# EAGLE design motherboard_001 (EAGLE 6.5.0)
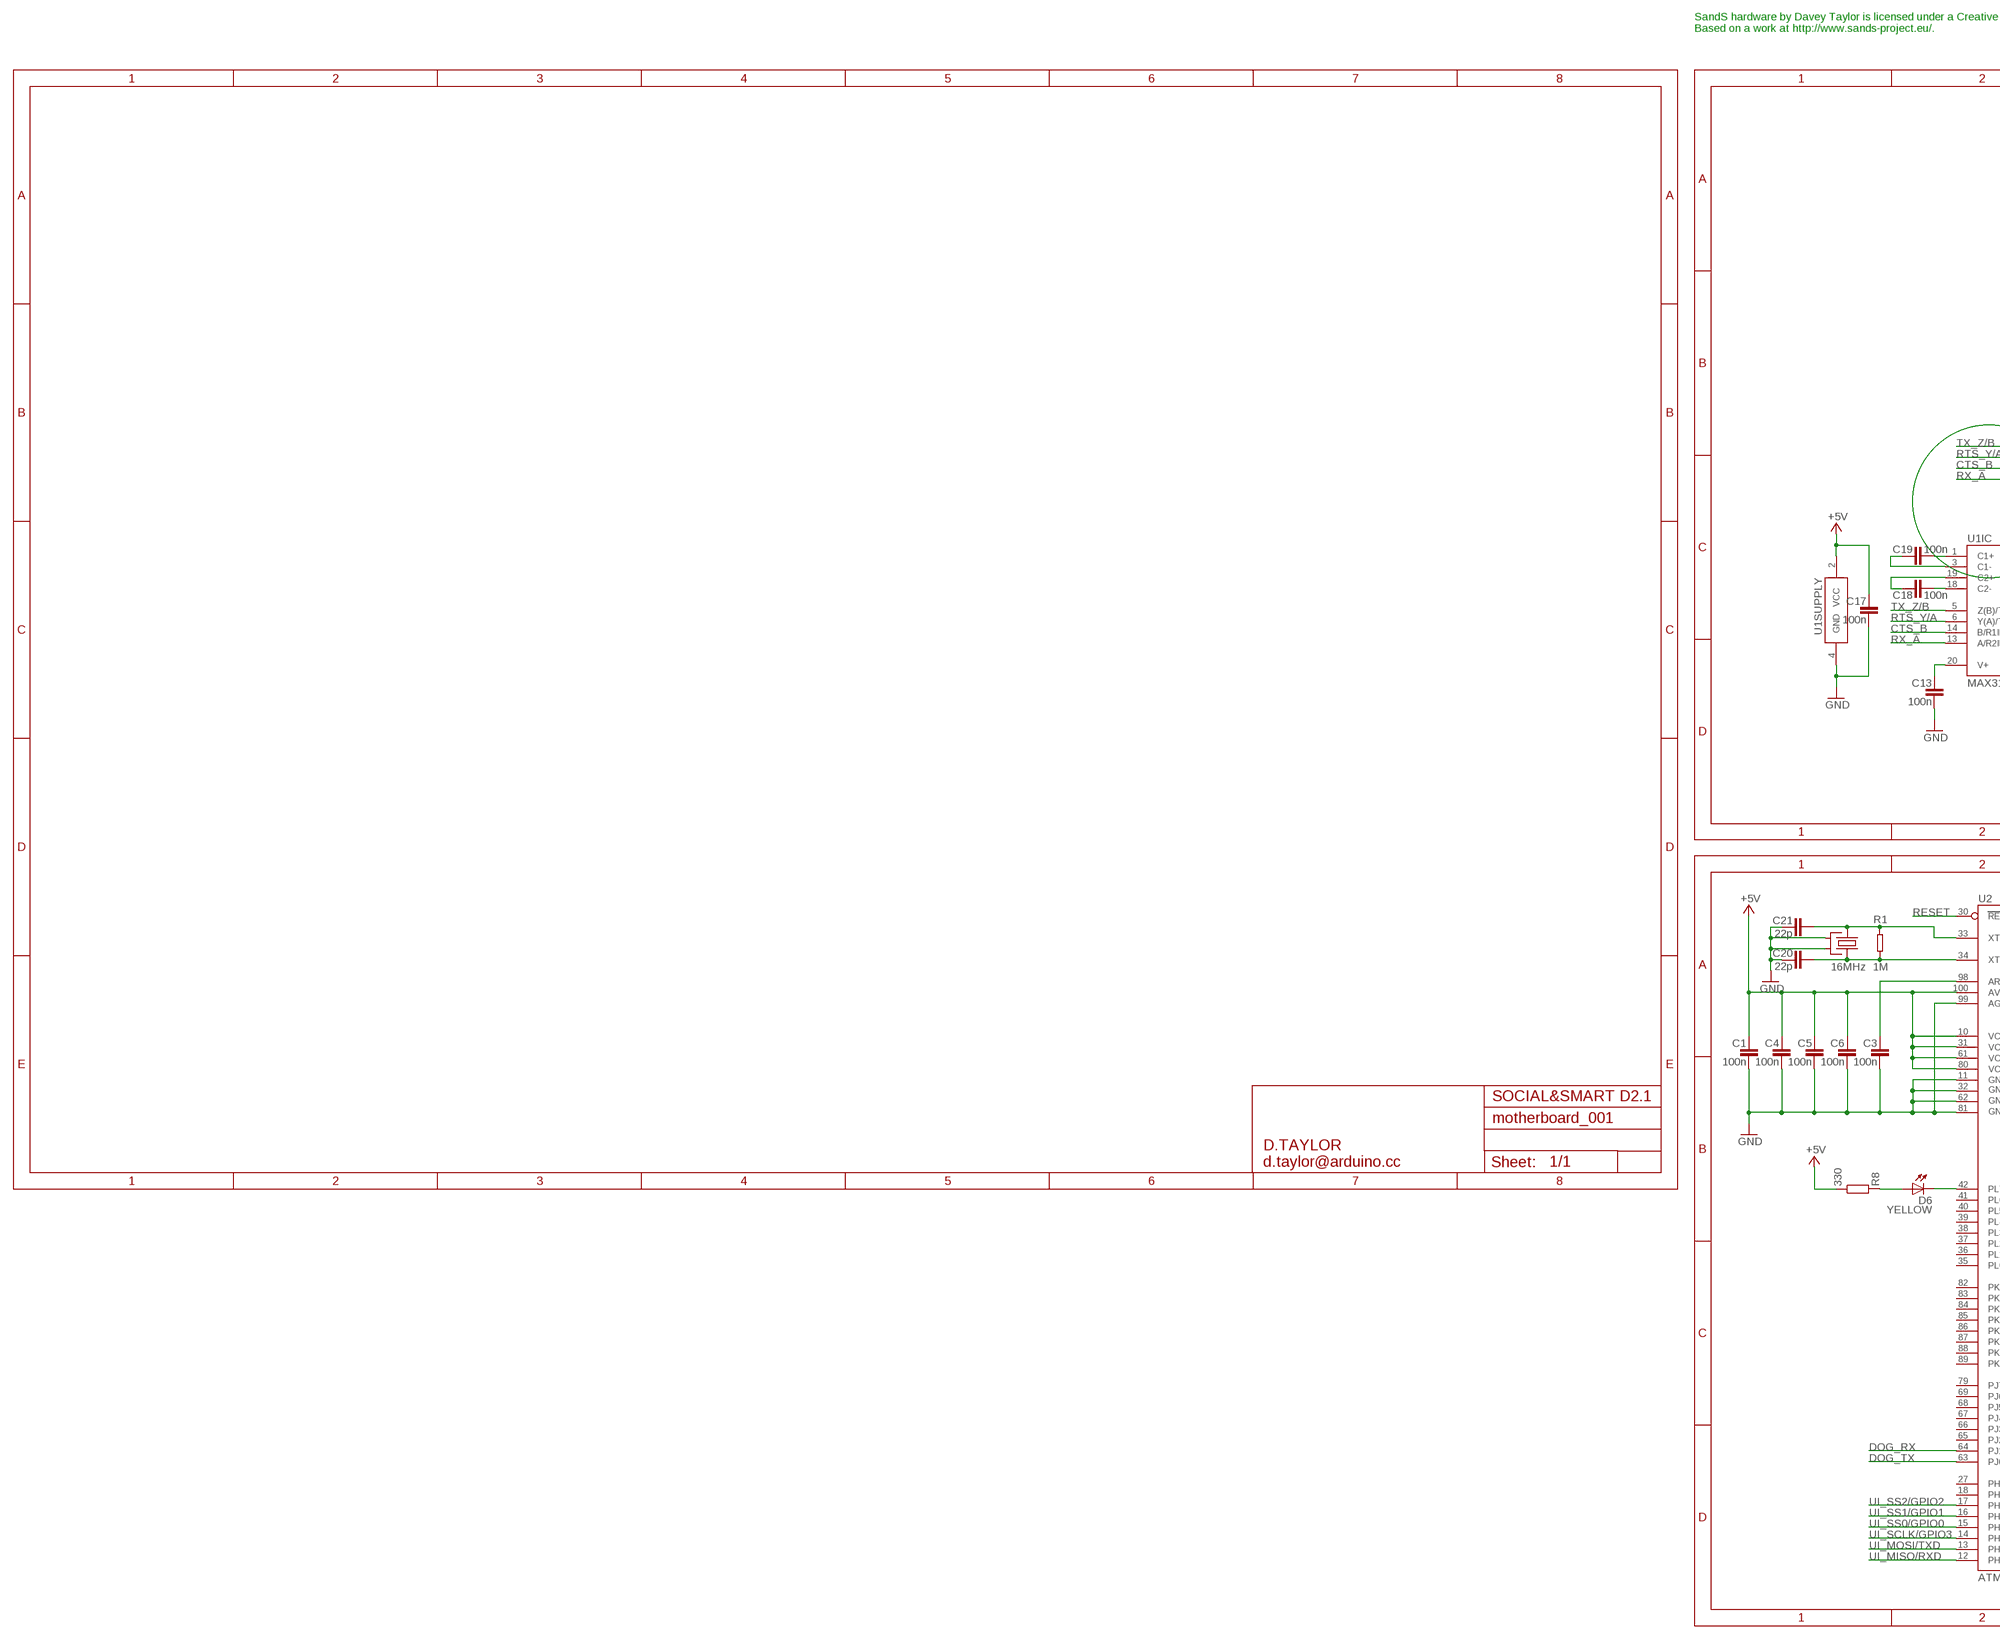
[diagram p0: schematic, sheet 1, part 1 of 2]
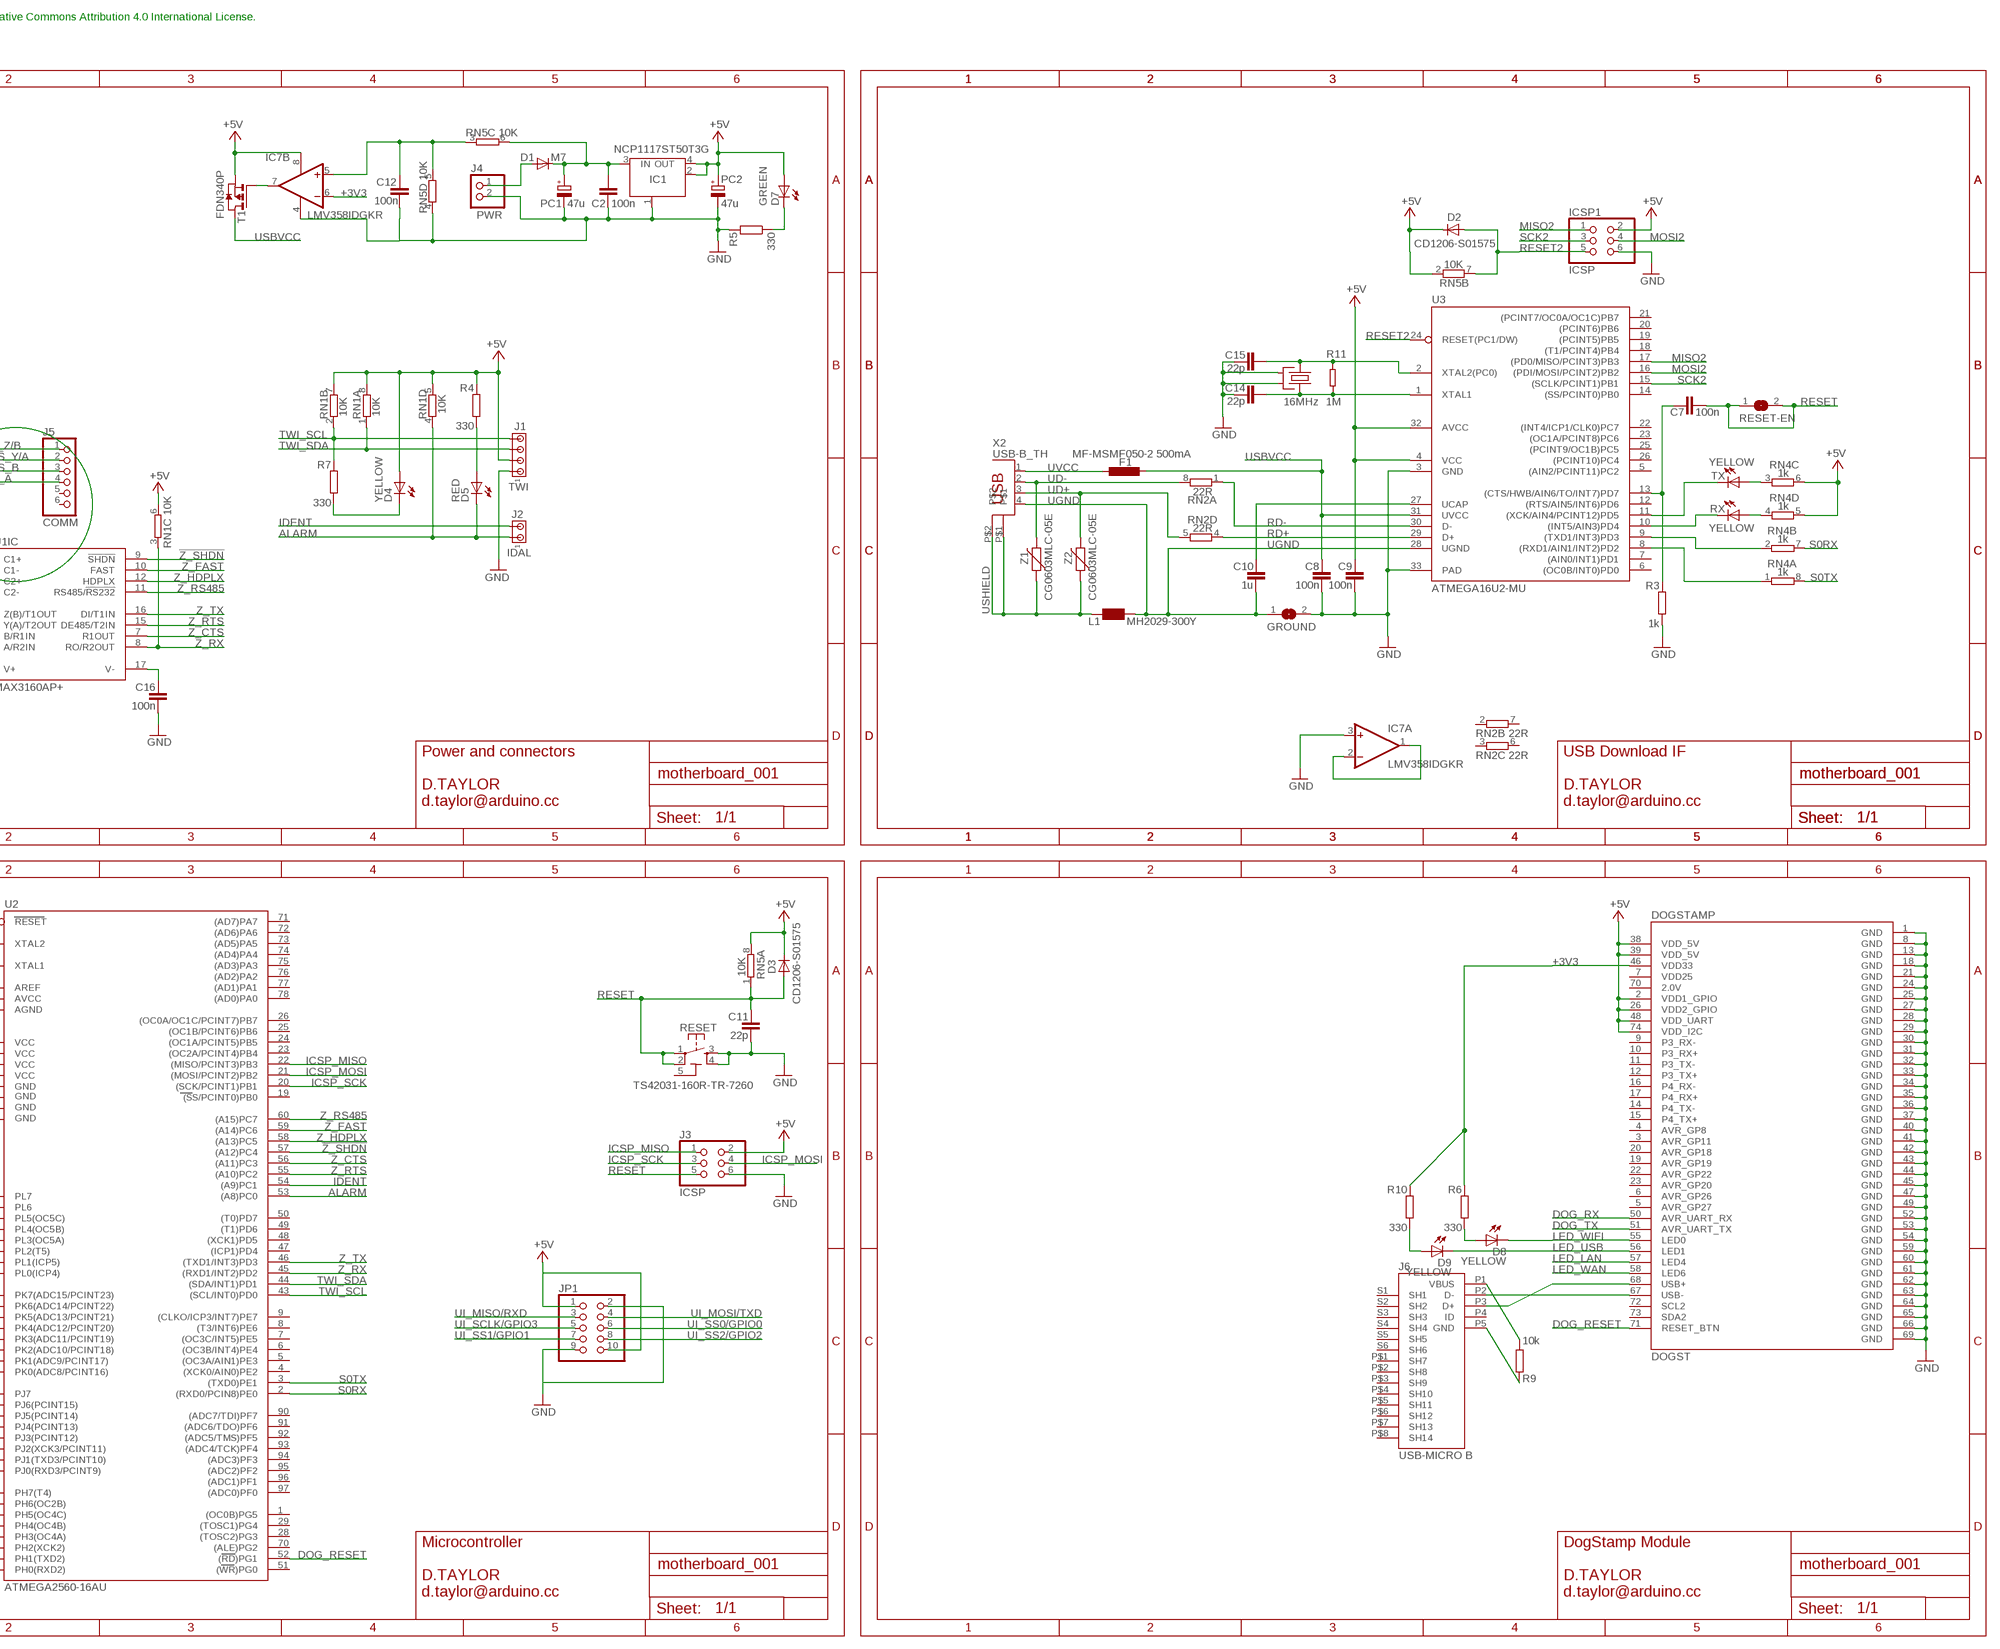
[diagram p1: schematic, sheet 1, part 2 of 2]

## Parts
C1  100n  C-EU0603-RND  [C0603-ROUND]
C2  100n  C-EU0603-RND  [C0603-ROUND]
C3  100n  C-EU0603-RND  [C0603-ROUND]
C4  100n  C-EU0603-RND  [C0603-ROUND]
C5  100n  C-EU0603-RND  [C0603-ROUND]
C6  100n  C-EU0603-RND  [C0603-ROUND]
C7  100n  C-EU0603-RND  [C0603-ROUND]
C8  100n  C-EU0603-RND  [C0603-ROUND]
C9  100n  C-EU0603-RND  [C0603-ROUND]
C10  1u  C-EU0603-RND  [C0603-ROUND]
C11  22p  C-EU0603-RND  [C0603-ROUND]
C12  100n  C-EU0603-RND  [C0603-ROUND]
C13  100n  C-EU0603-RND  [C0603-ROUND]
C14  22p  C-EU0603-RND  [C0603-ROUND]
C15  22p  C-EU0603-RND  [C0603-ROUND]
C16  100n  C-EU0603-RND  [C0603-ROUND]
C17  100n  C-EU0603-RND  [C0603-ROUND]
C18  100n  C-EU0603-RND  [C0603-ROUND]
C19  100n  C-EU0603-RND  [C0603-ROUND]
C20  22p  C-EU0603-RND  [C0603-ROUND]
C21  22p  C-EU0603-RND  [C0603-ROUND]
D1  M7  DIODE-SMB  [SMB]
D2  CD1206-S01575  DIODE-MINIMELF  [MINIMELF]
D3  CD1206-S01575  DIODE-MINIMELF  [MINIMELF]
D4  YELLOW  LEDCHIP-LED0805  [CHIP-LED0805]
D5  RED  LEDCHIP-LED0805  [CHIP-LED0805]
D6  YELLOW  LEDCHIP-LED0805  [CHIP-LED0805]
D7  GREEN  LEDCHIP-LED0805  [CHIP-LED0805]
D8  YELLOW  LEDCHIP-LED0805  [CHIP-LED0805]
D9  YELLOW  LEDCHIP-LED0805  [CHIP-LED0805]
DOGSTAMP  DOGST  [DOGST]
F1  MF-MSMF050-2 500mA  L-EUL1812  [L1812]
GROUND  SJ  [SJ]
IC1  NCP1117ST50T3G  MC33269ST-3.3T3  [SOT223]
IC7  LMV358IDGKR  LMV358MMX  [MSOP08]
ICSP1  ICSP  PINHD-2X3  [2X03]
J1  TWI  MTA04-100  [10X04MTA]
J2  IDAL  MTA02-100  [10X02MTA]
J3  ICSP  PINHD-2X3  [2X03]
J4  PWR  MKDS_1,5/2-5,08  [MKDS1,5/2-5,08]
J5  COMM  PINHD-1X6  [1X06]
J6  USB-MICRO B  MYCON2_USB-MINI-B  [CON2_USB_MICRO_B_AT]
JP1  PINHD-2X5  [2X05]
L1  MH2029-300Y  WE-CBF_0805  [0805]
PC1  47u  CPOL-EUD  [PANASONIC_D]
PC2  47u  CPOL-EUD  [PANASONIC_D]
R1  1M  R-EU_0603-RND  [R0603-ROUND]
R3  1k  R-EU_R0603  [R0603-ROUND]
R4  330  R-EU_R0603  [R0603-ROUND]
R5  330  R-EU_R0603  [R0603-ROUND]
R6  330  R-EU_R0603  [R0603-ROUND]
R7  330  R-EU_R0603  [R0603-ROUND]
R8  330  R-EU_R0603  [R0603-ROUND]
R9  10k  R-EU_R0603  [R0603-ROUND]
R10  330  R-EU_R0603  [R0603-ROUND]
R11  1M  R-EU_0603-RND  [R0603-ROUND]
RESET  TS42031-160R-TR-7260  TS42  [TS42]
RESET-EN  SJ  [SJ]
RN1  10K  4R-NCAT16  [CAT16]
RN2  22R  4R-NCAY16  [CAY16]
RN4  1k  4R-NCAY16  [CAY16]
RN5  10K  4R-NCAT16  [CAT16]
RX  YELLOW  LEDCHIP-LED0805  [CHIP-LED0805]
T1  FDN340P  PMOSSOT23  [SOT-23]
TX  YELLOW  LEDCHIP-LED0805  [CHIP-LED0805]
U1  MAX3160AP+  [SSOP20(G)]
U2  ATMEGA2560-16AU  ATMEGA25602560-16AU  [TQFP100]
U3  ATMEGA16U2-MU  [MLF32]
X1  16MHz  CRYSTAL2-KX7  [XTAL-3.2-2.5]
X2  USB-B_TH  PN61729  [PN61729]
X3  16MHz  CRYSTAL2-KX7  [XTAL-3.2-2.5]
Z1  CG0603MLC-05E  VARISTORCN0603  [CT/CN0603]
Z2  CG0603MLC-05E  VARISTORCN0603  [CT/CN0603]

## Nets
!Z_SHDN!: U1.9(IC:!SHDN!) U2.57((A12)PC4)
+3V3 [power]: DOGSTAMP.46(VDD33) IC7.6(B:-IN) R6.2 R10.2
+5V: C1.1 C4.1 C5.1 C6.1 C9.1 C17.1 D2.C D3.C D4.A D7.A DOGSTAMP.2(VDD1_GPIO) DOGSTAMP.26(VDD2_GPIO) DOGSTAMP.38(VDD_5V) DOGSTAMP.39(VDD_5V) DOGSTAMP.48(VDD_UART) DOGSTAMP.74(VDD_I2C) IC1.2(OUT) IC1.4(OUT) IC7.8(P:V+) ICSP1.2 J1.2 J3.2 JP1.1 JP1.10 PC2.+ R4.2 R8.1 RN1.5 RN1.6 RN1.7 RN1.8 RN4.5 RN4.6 RN5.2 RN5.8 T1.2(S) U1.2(SUPPLY:VCC) U2.10(VCC) U2.31(VCC1) U2.61(VCC2) U2.80(VCC3) U2.100(AVCC) U3.4(VCC) U3.32(AVCC)
ALARM: D5.C J2.1 RN1.4 U2.53((A8)PC0)
CMP: C12.2 IC7.5(B:+IN) RN5.3 RN5.5
CTS_B: J5.3 U1.14(IC:B/R1IN)
DOG_RESET: DOGSTAMP.71(RESET_BTN) U2.52((RD)PG1)
DOG_RX: DOGSTAMP.50(AVR_UART_RX) U2.64(PJ1(TXD3/PCINT10))
DOG_TX: DOGSTAMP.51(AVR_UART_TX) U2.63(PJ0(RXD3/PCINT9))
DTR: C7.1 R3.2 U3.13((CTS/HWB/AIN6/TO/INT7)PD7)
GATE_CMD: IC7.7(B:OUT) T1.3(G)
GND: C1.2 C2.2 C3.2 C4.2 C5.2 C6.2 C8.2 C9.2 C11.2 C12.1 C13.2 C14.2 C15.2 C16.2 C17.2 C20.2 C21.2 DOGSTAMP.1(GND) DOGSTAMP.8(GND) DOGSTAMP.13(GND) DOGSTAMP.18(GND) DOGSTAMP.21(GND) DOGSTAMP.24(GND) DOGSTAMP.25(GND) DOGSTAMP.27(GND) DOGSTAMP.28(GND) DOGSTAMP.29(GND) DOGSTAMP.30(GND) DOGSTAMP.31(GND) DOGSTAMP.32(GND) DOGSTAMP.33(GND) DOGSTAMP.34(GND) DOGSTAMP.35(GND) DOGSTAMP.36(GND) DOGSTAMP.37(GND) DOGSTAMP.40(GND) DOGSTAMP.41(GND) DOGSTAMP.42(GND) DOGSTAMP.43(GND) DOGSTAMP.44(GND) DOGSTAMP.45(GND) DOGSTAMP.47(GND) DOGSTAMP.49(GND) DOGSTAMP.52(GND) DOGSTAMP.53(GND) DOGSTAMP.54(GND) DOGSTAMP.59(GND) DOGSTAMP.60(GND) DOGSTAMP.61(GND) DOGSTAMP.62(GND) DOGSTAMP.63(GND) DOGSTAMP.64(GND) DOGSTAMP.65(GND) DOGSTAMP.66(GND) DOGSTAMP.69(GND) GROUND.2 IC1.1(GND/ADJ) IC7.3(A:+IN) IC7.4(P:V-) ICSP1.6 J1.1 J3.6 J4.2 JP1.2 JP1.9 PC1.- PC2.- R3.1 R5.2 RESET.3 RESET.4 RN5.4 U1.4(SUPPLY:GND) U2.11(GND) U2.32(GND1) U2.62(GND2) U2.81(GND3) U2.99(AGND) U3.3(GND) U3.33(PAD) X1.2(SH1) X1.4(SH2) X3.2(SH1) X3.4(SH2)
ICSP_MISO: J3.1 U2.22((MISO/PCINT3)PB3)
ICSP_MOSI: J3.4 U2.21((MOSI/PCINT2)PB2)
ICSP_SCK: J3.3 U2.20((SCK/PCINT1)PB1)
IDENT: J2.2 U2.54((A9)PC1)
LED_LAN: DOGSTAMP.57(LED4)
LED_USB: D9.C DOGSTAMP.56(LED1)
LED_WAN: DOGSTAMP.58(LED6)
LED_WIFI: D8.C DOGSTAMP.55(LED0)
M8RXD: RN4.2 U3.9((TXD1/INT3)PD3)
M8TXD: RN4.1 U3.8((RXD1/AIN1/INT2)PD2)
MISO2: ICSP1.1 U3.17((PD0/MISO/PCINT3)PB3)
MOSI2: ICSP1.4 U3.16((PDI/MOSI/PCINT2)PB2)
N$1: C3.1 U2.98(AREF)
N$2: IC7.1(A:OUT) IC7.2(A:-IN)
N$3: C14.1 R11.1 U3.1(XTAL1) X1.3(X2)
N$4: DOGSTAMP.68(USB+) J6.P3(D+)
N$5: D5.A R4.1
N$6: C19.2 U1.1(IC:C1+)
N$7: C18.2 U1.18(IC:C2-)
N$8: C18.1 U1.19(IC:C2+)
N$9: C19.1 U1.3(IC:C1-)
N$10: C13.1 U1.20(IC:V+)
N$11: C16.1 U1.17(IC:V-)
N$12: D7.C R5.1
N$13: D8.A R6.1
N$14: D4.C R7.1
N$15: D6.C U2.42(PL7)
N$16: D6.A R8.2
N$17: DOGSTAMP.67(USB-) J6.P2(D-)
N$18: J6.P1(VBUS) R9.1
N$19: J6.P5(GND) R9.2
N$20: D9.A R10.1
N$21: C20.1 R1.1 U2.34(XTAL1) X3.3(X2)
N$54: RN4.4 RX.A
N$55: RN4.3 TX.A
PWRIN [power]: D1.A J4.1
RD+: RN2.4 U3.29(D+)
RD-: RN2.1 U3.30(D-)
RESET: C7.2 C11.1 D3.A J3.5 RESET-EN.1 RESET-EN.2 RESET.1 RESET.2 RN5.1 U2.30(RESET)
RESET2: D2.A ICSP1.5 RN5.7 U3.24(RESET(PC1/DW))
RTS_Y/A: J5.2 U1.6(IC:Y(A)/T2OUT)
RX_A: J5.4 U1.13(IC:A/R2IN)
RXL: RX.C U3.10((INT5/AIN3)PD4)
S0RX: RN4.7 U2.2((RXD0/PCIN8)PE0)
S0TX: RN4.8 U2.3((TXD0)PE1)
SCK2: ICSP1.3 U3.15((SCLK/PCINT1)PB1)
TWI_SCL: J1.4 R7.2 RN1.2 U2.43((SCL/INT0)PD0)
TWI_SDA: J1.3 RN1.1 U2.44((SDA/INT1)PD1)
TX_Z/B: J5.1 U1.5(IC:Z(B)/T1OUT)
TXL: TX.C U3.11((XCK/AIN4/PCINT12)PD5)
UD+: RN2.5 X2.3 Z2.2
UD-: RN2.8 X2.2 Z1.2
UGND [gnd]: C10.2 GROUND.1 L1.1 U3.28(UGND) X2.4
UI_MISO/RXD: JP1.3 U2.12(PH0(RXD2))
UI_MOSI/TXD: JP1.4 U2.13(PH1(TXD2))
UI_SCLK/GPIO3: JP1.5 U2.14(PH2(XCK2))
UI_SS0/GPIO0: JP1.6 U2.15(PH3(OC4A))
UI_SS1/GPIO1: JP1.7 U2.16(PH4(OC4B))
UI_SS2/GPIO2: JP1.8 U2.17(PH5(OC4C))
USBVCC [power usb]: C8.1 F1.1 T1.1(D) U3.31(UVCC)
USHIELD [gnd]: L1.2 X2.P$1 X2.P$2 Z1.1 Z2.1
UVCC [power usb]: F1.2 X2.1
VIN [power]: C2.1 D1.C IC1.3(IN) PC1.+ RN5.6
VUCAP: C10.1 U3.27(UCAP)
XT1: C21.1 R1.2 U2.33(XTAL2) X3.1(X1)
XT2: C15.1 R11.2 U3.2(XTAL2(PC0)) X1.1(X1)
Z_CTS: U1.7(IC:R1OUT) U2.56((A11)PC3)
Z_FAST: U1.10(IC:FAST) U2.59((A14)PC6)
Z_HDPLX: U1.12(IC:HDPLX) U2.58((A13)PC5)
Z_RS485: U1.11(IC:RS485/!RS232!) U2.60((A15)PC7)
Z_RTS: U1.15(IC:DE485/T2IN) U2.55((A10)PC2)
Z_RX: RN1.3 U1.8(IC:RO/R2OUT) U2.45((RXD1/INT2)PD2)
Z_TX: U1.16(IC:DI/T1IN) U2.46((TXD1/INT3)PD3)
Unconnected: DOGSTAMP.3(AVR_GP11) DOGSTAMP.4(AVR_GP8) DOGSTAMP.5(AVR_GP27) DOGSTAMP.6(AVR_GP26) DOGSTAMP.7(VDD25) DOGSTAMP.9(P3_RX-) DOGSTAMP.10(P3_RX+) DOGSTAMP.11(P3_TX-) DOGSTAMP.12(P3_TX+) DOGSTAMP.14(P4_TX-) DOGSTAMP.15(P4_TX+) DOGSTAMP.16(P4_RX-) DOGSTAMP.17(P4_RX+) DOGSTAMP.19(AVR_GP19) DOGSTAMP.20(AVR_GP18) DOGSTAMP.22(AVR_GP22) DOGSTAMP.23(AVR_GP20) DOGSTAMP.70(2.0V) DOGSTAMP.72(SCL2) DOGSTAMP.73(SDA2) J5.5 J5.6 J6.P4(ID) J6.P$1(SH7) J6.P$2(SH8) J6.P$3(SH9) J6.P$4(SH10) J6.P$5(SH11) J6.P$6(SH12) J6.P$7(SH13) J6.P$8(SH14) J6.S1(SH1) J6.S2(SH2) J6.S3(SH3) J6.S4(SH4) J6.S5(SH5) J6.S6(SH6) RN2.2 RN2.3 RN2.6 RN2.7 U2.1((OC0B)PG5) U2.4((XCK0/AIN0)PE2) U2.5((OC3A/AIN1)PE3) U2.6((OC3B/INT4)PE4) U2.7((OC3C/INT5)PE5) U2.8((T3/INT6)PE6) U2.9((CLKO/ICP3/INT7)PE7) U2.18(PH6(OC2B)) U2.19((SS/PCINT0)PB0) U2.23((OC2A/PCINT4)PB4) U2.24((OC1A/PCINT5)PB5) U2.25((OC1B/PCINT6)PB6) U2.26((OC0A/OC1C/PCINT7)PB7) U2.27(PH7(T4)) U2.28((TOSC2)PG3) U2.29((TOSC1)PG4) U2.35(PL0(ICP4)) U2.36(PL1(ICP5)) U2.37(PL2(T5)) U2.38(PL3(OC5A)) U2.39(PL4(OC5B)) U2.40(PL5(OC5C)) U2.41(PL6) U2.47((ICP1)PD4) U2.48((XCK1)PD5) U2.49((T1)PD6) U2.50((T0)PD7) U2.51((WR)PG0) U2.65(PJ2(XCK3/PCINT11)) U2.66(PJ3(PCINT12)) U2.67(PJ4(PCINT13)) U2.68(PJ5(PCINT14)) U2.69(PJ6(PCINT15)) U2.70((ALE)PG2) U2.71((AD7)PA7) U2.72((AD6)PA6) U2.73((AD5)PA5) U2.74((AD4)PA4) U2.75((AD3)PA3) U2.76((AD2)PA2) U2.77((AD1)PA1) U2.78((AD0)PA0) U2.79(PJ7) U2.82(PK7(ADC15/PCINT23)) U2.83(PK6(ADC14/PCINT22)) U2.84(PK5(ADC13/PCINT21)) U2.85(PK4(ADC12/PCINT20)) U2.86(PK3(ADC11/PCINT19)) U2.87(PK2(ADC10/PCINT18)) U2.88(PK1(ADC9/PCINT17)) U2.89(PK0(ADC8/PCINT16)) U2.90((ADC7/TDI)PF7) U2.91((ADC6/TDO)PF6) U2.92((ADC5/TMS)PF5) U2.93((ADC4/TCK)PF4) U2.94((ADC3)PF3) U2.95((ADC2)PF2) U2.96((ADC1)PF1) U2.97((ADC0)PF0) U3.5((AIN2/PCINT11)PC2) U3.6((OC0B/INT0)PD0) U3.7((AIN0/INT1)PD1) U3.12((RTS/AIN5/INT6)PD6) U3.14((SS/PCINT0)PB0) U3.18((T1/PCINT4)PB4) U3.19((PCINT5)PB5) U3.20((PCINT6)PB6) U3.21((PCINT7/OC0A/OC1C)PB7) U3.22((INT4/ICP1/CLK0)PC7) U3.23((OC1A/PCINT8)PC6) U3.25((PCINT9/OC1B)PC5) U3.26((PCINT10)PC4)

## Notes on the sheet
- SandS hardware by Davey Taylor is licensed under a Creative Commons Attribution 4.0 International License.
  Based on a work at http://www.sands-project.eu/.
- Power and connectors
  
  D.TAYLOR
  d.taylor@arduino.cc
- USB Download IF
  
  D.TAYLOR
  d.taylor@arduino.cc
- SOCIAL&SMART D2.1
- D.TAYLOR
  d.taylor@arduino.cc
- Microcontroller
  
  D.TAYLOR
  d.taylor@arduino.cc
- DogStamp Module
  
  D.TAYLOR
  d.taylor@arduino.cc

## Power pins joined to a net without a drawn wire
5-GND: RESET.5(5-GND)

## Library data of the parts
C1-C21 = SmartPrj:C-EU: CAPACITOR, European symbol
D1-D3 = diode:DIODE-: DIODE
D4-D9 RX TX = led:LED: LED
DOGSTAMP = d_taylor:DOGST
F1 = rcl:L-EU: INDUCTOR, European symbol
GROUND RESET-EN = jumper:SJ: SMD solder JUMPER
IC1 = linear:MC33269ST*: Adjustable Output Low Dropout Voltage Regulator 800 mA Source: http://www.onsemi.com/pub/Collateral/MC33269-D.PDF
IC7 = linear:LMV358?*: Dual General Purpose, Low Voltage, Rail-to-Rail Output Operational Amplifiers Source: http://www.national.com/mpf/LM/LMV321.html http://www.national.com/dt/lmv_qual.pdf
ICSP1 = SmartPrj:PINHD-2X3: PIN HEADER
J1 = con-amp:MTA04-100: AMP connector
J2 = con-amp:MTA02-100: AMP connector
J3 = pinhead:PINHD-2X3: PIN HEADER
J4 = d_taylor:MKDS_1,5/2-5,08: Screw terminal header
J5 = pinhead:PINHD-1X6: PIN HEADER
J6 = SmartPrj:MYCON2_USB-MINI-B
JP1 = pinhead:PINHD-2X5: PIN HEADER
L1 = wuerth-elektronik:WE-CBF: SMD EMI Suppression Ferrite Beads
PC1 PC2 = rcl:CPOL-EU: POLARIZED CAPACITOR, European symbol
R1 R11 = d_taylor:R-EU_: RESISTOR, European symbol
R3-R10 = SmartPrj:R-EU_: RESISTOR, European symbol
RESET = SmartPrj:TS42: TS42 Dongnan Electronics Tact switch VDC 12V - 50mA
RN1 RN2 RN4 RN5 = resistor-dil:4R-N: Array Chip Resistor Source: RS Component / Phycomp; OC_FARNELL: unknown; OC_NEWARK: unknown
T1 = zetex:PMOSSOT23: MOS FET; OC_FARNELL: unknown; OC_NEWARK: unknown
U1 = d_taylor:MAX3160*AP+
U2 = SmartPrj:ATMEGA2560: MICROCONTROLLER 64/128/256 Kbytes FLASH 4 Kbytes EEPROM 8 Kbytes SRAM 86 General Purpose I/O pins 12-channels16-bit PWM 4 x Serial USARTs 16-channels 10-bit A/D
U3 = SmartPrj:ATMEGA16U2-
X1 X3 = d_taylor:CRYSTAL2: KX7 SMD crystal
X2 = SmartPrj:PN61729: BERG USB connector
Z1 Z2 = varistor:VARISTOR: VARISTOR

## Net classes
0 default: width 0.203 mm, drill 0.406 mm, clearance 0.203 mm
1 power: width 0.61 mm, drill 0.406 mm, clearance 0.203 mm
2 gnd: width 0.305 mm, drill 0.406 mm, clearance 0.203 mm
3 power usb: width 0.508 mm, drill 0.406 mm, clearance 0.203 mm

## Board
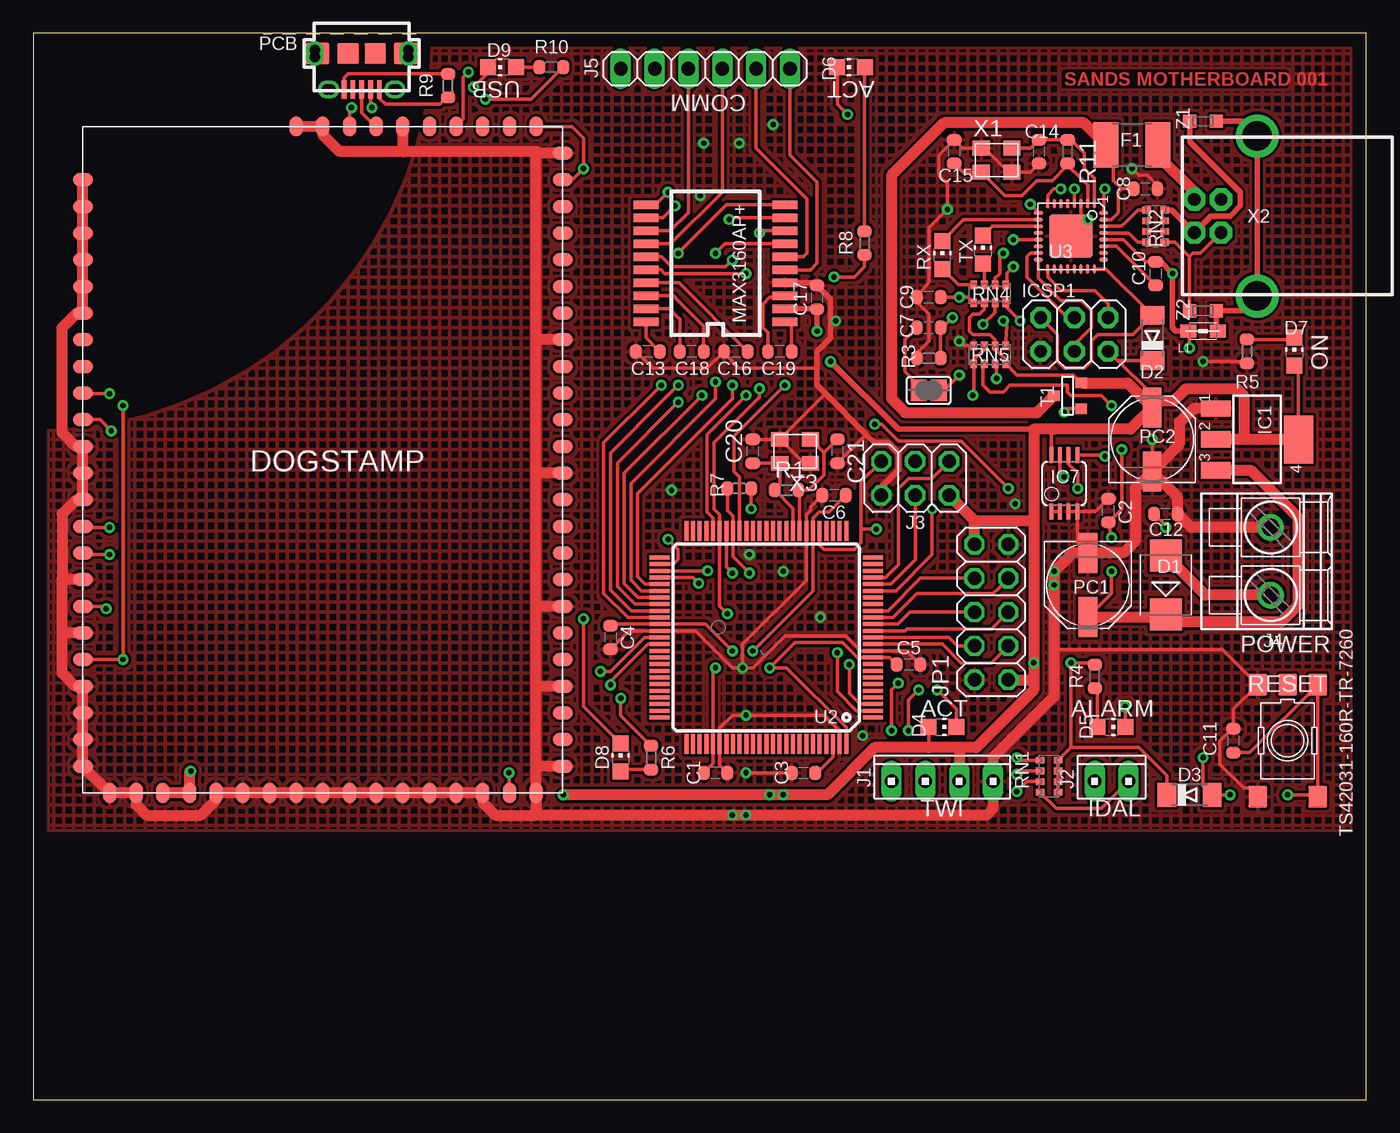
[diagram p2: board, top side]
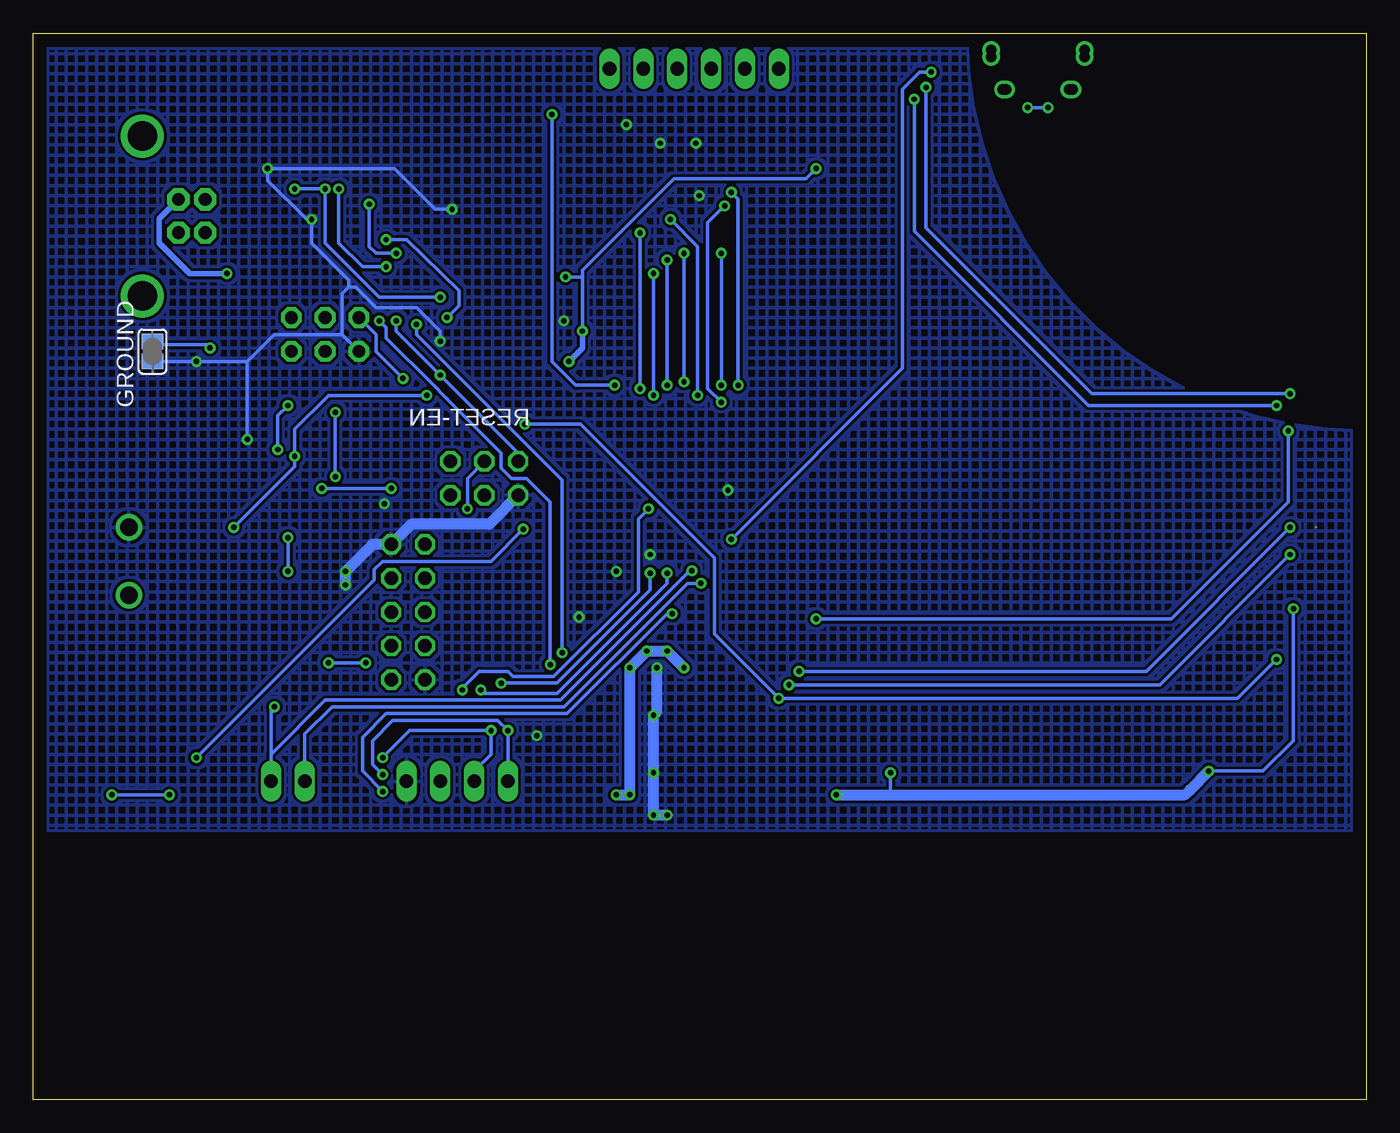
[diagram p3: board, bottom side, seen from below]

Size 100 x 80 mm. Coordinates in mm from the lower left corner, seen from the top.
Outline: 0,0 100,0 100,80 0,80 0,0
Copper layers (1*16): Top 0.035mm / dielectric 1.5mm / Bottom 0.035mm
Design rules "default *": minimum track width 10mil, minimum drill 16mil, track to track 8mil, track to pad 8mil, pad to pad 8mil, via to via 8mil, smd to smd 8mil, copper to edge 40mil, drill to drill 8mil, minimum pad ring 10mil, minimum via ring 8mil, stop-mask expansion 4mil, vias tented up to drill 0mil, thermal gap 10mil

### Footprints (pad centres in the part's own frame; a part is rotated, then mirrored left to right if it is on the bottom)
C0603-ROUND = smd 0.898 x 1.1: 1 -0.889,0; 2 0.889,0
SMB = smd 2.4 x 2.4: A 2.2,0; C -2.2,0
MINIMELF = smd 1.4 x 1.8: A 1.7,0; C -1.7,0
CHIP-LED0805 = smd 1.2 x 1.2: A 0,-1.05; C 0,1.05
DOGST = smd 1 x 1.5: 1 -23,18; 2 -21,18; 3 -19,18; 4 -17,18; 5 -15,18; 6 -13,18; 7 -11,18; 8 -9,18; 9 -7,18; 10 -5,18; 11 -3,18; 12 -1,18; 13 1,18; 14 3,18; 15 5,18; 16 7,18; 17 9,18; 18 11,18; 19 13,18; 20 15,18; 21 17,18; 22 19,18; 23 21,18; 24 23,18; 42 23,-18; 43 21,-18; 44 19,-18; 45 17,-18; 46 15,-18; 47 13,-18; 48 11,-18; 49 9,-18; 50 7,-18; 51 5,-18; 52 3,-18; 53 1,-18; 54 -1,-18; 55 -3,-18; 56 -5,-18; 57 -7,-18; 58 -9,-18; 59 -11,-18; 60 -13,-18; 61 -15,-18; 62 -17,-18; 63 -19,-18; 64 -21,-18 | smd 1.5 x 1: 25 25,16; 26 25,14; 27 25,12; 28 25,10; 29 25,8; 30 25,6; 31 25,4; 32 25,2; 33 25,0; 34 25,-2; 35 25,-4; 36 25,-6; 37 25,-8; 38 25,-10; 39 25,-12; 40 25,-14; 41 25,-16; 65 -25,-2; 66 -25,0; 67 -25,2; 68 -25,4; 69 -25,6; 70 -25,8; 71 -25,10; 72 -25,12; 73 -25,14; 74 -25,16
L1812 = smd 1.9 x 3.4: 1 -1.95,0; 2 1.95,0
SJ = smd 1.168 x 1.6: 1 -0.762,0; 2 0.762,0
SOT223 = smd 1.219 x 2.235: 1 -2.311,-3.099; 2 0,-3.099; 3 2.311,-3.099 | smd 3.6 x 2.2: 4 0,3.099
MSOP08 = smd 0.3 x 1.2: 1 -0.976,-2.113; 2 -0.326,-2.113; 3 0.324,-2.113; 4 0.974,-2.113; 5 0.974,2.112; 6 0.324,2.112; 7 -0.326,2.112; 8 -0.976,2.112
2X03 = drill 0.95 pad 1.55 octagon: 1 -2.54,-1.27; 2 -2.54,1.27; 3 0,-1.27; 4 0,1.27; 5 2.54,-1.27; 6 2.54,1.27
10X04MTA = drill 1.016 long: 1 3.81,0; 2 1.27,0; 3 -1.27,0; 4 -3.81,0
10X02MTA = drill 1.016 long: 1 1.27,0; 2 -1.27,0
2X03' = drill 1.016 octagon: 1 -2.54,-1.27; 2 -2.54,1.27; 3 0,-1.27; 4 0,1.27; 5 2.54,-1.27; 6 2.54,1.27
MKDS1,5/2-5,08 = drill 1.3 pad 2: 1 -2.54,0; 2 2.54,0
1X06 = drill 1.016 long: 1 -6.35,0; 2 -3.81,0; 3 -1.27,0; 4 1.27,0; 5 3.81,0; 6 6.35,0
CON2_USB_MICRO_B_AT = smd 0.406 x 1.346: P1 -1.321,2.692; P2 -0.66,2.692; P3 0,2.692; P4 0.66,2.692; P5 1.321,2.692 | drill 0.8 pad 1.27: P$1 -2.616,2.692 | drill 0.8 pad 1.245: P$2 -2.362,2.692; P$7 2.362,2.692; P$8 2.616,2.692 | drill 0.8 pad 1.143: P$3 -3.505,-0.254; P$4 -3.505,0.254; P$5 3.505,0.254; P$6 3.505,-0.254 | smd 1.778 x 1.651: S1 -3.302,0; S2 3.302,0 | smd 1.524 x 1.27: S3 -2.489,2.692; S4 2.489,2.692 | smd 1.626 x 1.524: S5 -1.016,0; S6 1.016,0
2X05 = drill 1.016 octagon: 1 -5.08,-1.27; 2 -5.08,1.27; 3 -2.54,-1.27; 4 -2.54,1.27; 5 0,-1.27; 6 0,1.27; 7 2.54,-1.27; 8 2.54,1.27; 9 5.08,-1.27; 10 5.08,1.27
0805 = smd 1.2 x 1: 1 -1.1,0; 2 1.1,0
PANASONIC_D = smd 3 x 1.4: + 2.4,0; - -2.4,0
R0603-ROUND = smd 0.898 x 1.1: 1 -0.889,0; 2 0.889,0
TS42 = smd 1.6 x 1.4: 1 -4.2,2.25; 2 4.2,2.25; 3 -4.2,-2.25; 4 4.2,-2.25; 5 -4.2,0
CAT16 = smd 0.5 x 0.65: 1 -1.2,-0.675; 2 -0.4,-0.675; 3 0.4,-0.675; 4 1.2,-0.675; 5 1.2,0.675; 6 0.4,0.675; 7 -0.4,0.675; 8 -1.2,0.675
CAY16 = smd 0.5 x 0.65: 1 -1.2,-0.675; 2 -0.4,-0.675; 3 0.4,-0.675; 4 1.2,-0.675; 5 1.2,0.675; 6 0.4,0.675; 7 -0.4,0.675; 8 -1.2,0.675
SOT-23 = smd 0.787 x 0.889: 1 0.025,-1.016; 2 -0.94,1.016; 3 0.991,1.016
SSOP20(G) = smd 0.63 x 1.875: 1 -4.388,-5.213; 2 -3.413,-5.213; 3 -2.438,-5.213; 4 -1.462,-5.213; 5 -0.487,-5.213; 6 0.487,-5.213; 7 1.462,-5.213; 8 2.438,-5.213; 9 3.413,-5.213; 10 4.388,-5.213; 11 4.388,5.213; 12 3.413,5.213; 13 2.438,5.213; 14 1.462,5.213; 15 0.487,5.213; 16 -0.487,5.213; 17 -1.462,5.213; 18 -2.438,5.213; 19 -3.413,5.213; 20 -4.388,5.213
TQFP100 = smd 1.5 x 0.3: 1 -8,6; 2 -8,5.5; 3 -8,5; 4 -8,4.5; 5 -8,4; 6 -8,3.5; 7 -8,3; 8 -8,2.5; 9 -8,2; 10 -8,1.5; 11 -8,1; 12 -8,0.5; 13 -8,0; 14 -8,-0.5; 15 -8,-1; 16 -8,-1.5; 17 -8,-2; 18 -8,-2.5; 19 -8,-3; 20 -8,-3.5; 21 -8,-4; 22 -8,-4.5; 23 -8,-5; 24 -8,-5.5; 25 -8,-6; 51 8,-6; 52 8,-5.5; 53 8,-5; 54 8,-4.5; 55 8,-4; 56 8,-3.5; 57 8,-3; 58 8,-2.5; 59 8,-2; 60 8,-1.5; 61 8,-1; 62 8,-0.5; 63 8,0; 64 8,0.5; 65 8,1; 66 8,1.5; 67 8,2; 68 8,2.5; 69 8,3; 70 8,3.5; 71 8,4; 72 8,4.5; 73 8,5; 74 8,5.5; 75 8,6 | smd 0.3 x 1.5: 26 -6,-8; 27 -5.5,-8; 28 -5,-8; 29 -4.5,-8; 30 -4,-8; 31 -3.5,-8; 32 -3,-8; 33 -2.5,-8; 34 -2,-8; 35 -1.5,-8; 36 -1,-8; 37 -0.5,-8; 38 0,-8; 39 0.5,-8; 40 1,-8; 41 1.5,-8; 42 2,-8; 43 2.5,-8; 44 3,-8; 45 3.5,-8; 46 4,-8; 47 4.5,-8; 48 5,-8; 49 5.5,-8; 50 6,-8; 76 6,8; 77 5.5,8; 78 5,8; 79 4.5,8; 80 4,8; 81 3.5,8; 82 3,8; 83 2.5,8; 84 2,8; 85 1.5,8; 86 1,8; 87 0.5,8; 88 0,8; 89 -0.5,8; 90 -1,8; 91 -1.5,8; 92 -2,8; 93 -2.5,8; 94 -3,8; 95 -3.5,8; 96 -4,8; 97 -4.5,8; 98 -5,8; 99 -5.5,8; 100 -6,8
MLF32 = smd 0.7 x 0.28: 1 -2.45,1.75; 2 -2.45,1.25; 3 -2.45,0.75; 4 -2.45,0.25; 5 -2.45,-0.25; 6 -2.45,-0.75; 7 -2.45,-1.25; 8 -2.45,-1.75; 17 2.45,-1.75; 18 2.45,-1.25; 19 2.45,-0.75; 20 2.45,-0.25; 21 2.45,0.25; 22 2.45,0.75; 23 2.45,1.25; 24 2.45,1.75 | smd 0.28 x 0.7: 9 -1.75,-2.45; 10 -1.25,-2.45; 11 -0.75,-2.45; 12 -0.25,-2.45; 13 0.25,-2.45; 14 0.75,-2.45; 15 1.25,-2.45; 16 1.75,-2.45; 25 1.75,2.45; 26 1.25,2.45; 27 0.75,2.45; 28 0.25,2.45; 29 -0.25,2.45; 30 -0.75,2.45; 31 -1.25,2.45; 32 -1.75,2.45 | smd 3.254 x 3.254: 33 0,0
XTAL-3.2-2.5 = smd 1.3 x 1.1: 1 -1.15,-0.9; 2 1.15,-0.9; 3 1.15,0.9; 4 -1.15,0.9
PN61729 = drill 0.95 pad 1.676 octagon: 1 1.25,4.71; 2 -1.25,4.71; 3 -1.25,2.71; 4 1.25,2.71 | drill 2.2: P$1 -6,0; P$2 6,0
CT/CN0603 = smd 1 x 1: 1 -1,0; 2 1,0

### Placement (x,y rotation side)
C1  51.18,24.51 0 top
C2  80.64,44.2 90 top
C3  57.78,24.51 180 top
C4  43.31,34.67 270 top
C5  65.66,32.64 0 top
C6  60.07,45.34 180 top
C7  67.18,57.91 180 top
C8  83.44,68.33 0 top
C9  67.18,60.2 180 top
C10  84.2,61.98 90 top
C11  90.04,26.92 90 top
C12  84.96,43.94 180 top
C13  46.1,56.13 180 top
C14  75.44,71.12 270 top
C15  69.09,71.12 90 top
C16  52.7,56.13 180 top
C17  58.8,60.2 90 top
C18  49.4,56.13 0 top
C19  56.01,56.13 0 top
C20  53.98,48.64 90 top
C21  60.33,48.64 270 top
D1  84.96,38.61 90 top
D2  83.95,57.15 90 top
D3  86.74,22.86 0 top
D4  68.2,27.94 270 top
D5  80.9,27.94 270 top
D6  61.34,77.47 90 top
D7  94.61,56.13 0 top
D8  44.07,25.65 0 top
D9  35.18,77.47 90 top
DOGSTAMP  21.72,48.01 270 top
F1  82.42,71.63 0 top
GROUND  91.06,56.13 270 bottom
IC1  91.82,49.53 270 top
IC7  77.34,46.23 0 top
ICSP1  78.11,57.4 180 top
J1  68.2,23.88 0 top
J2  80.9,23.88 0 top
J3  ICSP  [2X03']  66.17,46.61 180 top
J4  92.84,40.39 90 top
J5  50.42,77.34 180 top
J6  24.64,78.49 180 top
JP1  71.88,36.58 90 top
L1  87.76,57.66 0 top
PC1  79.12,38.61 270 top
PC2  83.95,49.53 90 top
R1  56.52,45.72 0 top
R3  67.18,55.63 0 top
R4  79.63,31.75 90 top
R5  91.06,56.13 270 top
R6  46.35,25.65 90 top
R7  52.96,45.85 180 top
R8  62.36,64.26 90 top
R9  31.11,76.07 90 top
R10  38.86,77.47 0 top
R11  77.6,71.12 270 top
RESET  94.11,26.92 270 top
RESET-EN  67.18,53.21 0 top
RN1  76.2,24.26 270 top
RN2  84.2,65.53 270 top
RN4  71.75,60.45 180 top
RN5  71.75,55.88 180 top
RX  68.2,63.37 0 top
T1  77.6,52.83 270 top
TX  71.25,63.75 0 top
U1  51.18,62.74 90 top
U2  54.99,34.67 180 top
U3  77.85,64.77 270 top
X1  72.26,70.48 0 top
X2  91.82,66.29 90 top
X3  57.15,48.64 180 top
Z1  87.76,73.41 180 top
Z2  87.76,59.18 180 top

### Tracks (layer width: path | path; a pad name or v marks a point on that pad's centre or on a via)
!Z_SHDN!  (via drill 0.41)
  Top 0.254: v52.2,66.04 52.31,66.15 54.24,66.15 U1.9 | v50.16,52.83 44.32,46.99 44.32,38.73 45.39,37.67 U2.57
  Bottom 0.254: v52.2,66.04 50.16,64.01 50.16,61.47 v50.16,52.83
+3V3  (via drill 0.41)
  Top 0.254: DOGSTAMP.46 6.46,33.01 v6.73,33.02 v6.73,52.07 | v78.36,45.85 78.36,46.99 77.67,47.68 IC7.6 | R6.2 44.07,28.83 v44.07,30.1 | v33.91,75.06 37.34,75.06 R10.2 | v63.12,50.67 63.63,50.67 64.9,49.4 69.6,49.4 v73.15,45.85
  Bottom 0.254: v6.73,33.02 9.65,30.1 v44.07,30.1 48.9,34.92 48.9,40.64 58.93,50.67 v63.12,50.67 | v73.15,45.85 v78.36,45.85 | v6.73,52.07 20.83,52.07 33.91,65.15 v33.91,75.06
+5V  (via drill 0.41)
  Top 0.254: v78.11,68.33 U3.4 | U3.32 80.3,68.49 v80.39,68.33 | C9.1 v69.47,60.2 70.13,60.2 RN4.5 RN4.6 71.36,59.29 70.99,58.93 70.48,58.93 70.23,58.67 70.23,57.66 70.48,57.4 71.75,57.4 72.16,57 RN5.2 72.16,56.24 72.14,56.26 72.95,55.57 RN5.8 | PC2.+ 84.45,52.44 ICSP1.2 81.33,55.45 D2.C | RN5.8 72.85,55.06 | IC7.8 76.37,50.08 76.58,50.29 | T1.2 78.03,54.36 74.04,54.36 73.8,54.36 RN5.8 | 76.88,25.44 RN1.8 76.88,25.44 | 76.88,25.44 RN1.7 RN1.6 RN1.5 | 58.78,59.33 C17.1 | 76.88,25.44 77.85,26.42 | 77.85,26.42 82.93,26.42 85.04,24.31 D3.C | 77.85,26.42 v77.85,32.77 79.5,32.77 R4.2 | v51.18,32.38 50.99,32.2 U2.80 50.99,25.21 C1.1 | v52.45,33.66 50.44,35.67 U2.61 43.7,35.67 C4.1 | v53.98,33.66 58.49,38.17 U2.31 58.49,43.63 58.93,44.07 59.69,44.07 C6.1 | U2.100 60.99,27.91 56.52,32.38 v55.24,32.38 56.03,33.17 57.15,34.29 60.71,34.29 61.83,33.17 U2.10 64.24,33.17 C5.1 | v5.46,36.83 5.29,37.01 DOGSTAMP.48 | DOGSTAMP.74 40.41,73.01 41.27,72.14 41.27,71.12 | 41.27,71.12 v41.27,69.85 | v41.27,69.85 40.51,69.09 39.8,69.09 DOGSTAMP.2 | v41.27,69.85 41.27,71.12 | D7.A 94.92,54.78 IC1.4 | D4.A 67.18,27.91 67.18,26.42 | R8.1 62.36,62.87 62.36,62.48 61.59,61.72 v60.07,61.72 | DOGSTAMP.26 35.69,23.37 v35.69,24.51
  Top 0.406: U1.2 58.78,59.33 | 75.06,50.29 64.9,50.29 v59.82,55.37 | v58.8,57.66 C17.1
  Top 0.813: IC1.4 90.81,49.53 | 90.81,49.53 IC1.2 | 84.45,52.44 85.58,52.44 86.23,53.09 86.49,53.34 90.3,53.34 90.81,52.83 90.81,49.53 | T1.2 82.11,53.77 PC2.+ 82.31,50.29 76.58,50.29 76.33,50.29 75.06,50.29 75.06,43.43 | 75.06,43.43 v75.06,32.77 75.06,31.62 | 75.06,31.62 75.06,30.73 70.74,26.42 69.47,26.42 | 69.47,26.42 J1.2 69.47,23.37 | 69.47,26.42 67.18,26.42 63.12,26.42 59.56,22.86 v56.26,22.86 v55.24,22.86 v39.75,22.86 | v11.81,24.64 11.72,24.54 DOGSTAMP.38 DOGSTAMP.39 | JP1.10 70.61,43.43 | 70.61,43.43 J3.2 | 70.61,43.43 75.06,43.43 | JP1.1 74.93,31.5 75.06,31.62
  Bottom 0.254: v80.39,68.33 v78.11,68.33 78.11,64.26 74.04,60.2 v69.47,60.2 | v75.06,32.77 v77.85,32.77 | v11.81,24.64 7.75,24.64 5.46,26.92 v5.46,36.83 | v58.8,57.66 58.8,61.72 | 58.8,61.72 58.8,62.23 51.94,69.09 42.04,69.09 v41.27,69.85 | v60.07,61.72 58.8,61.72 | v35.69,24.51 35.69,22.86
  Bottom 0.406: v59.82,55.37 58.8,56.39 v58.8,57.66
  Bottom 0.813: v39.75,22.86 35.69,22.86 13.59,22.86 13.21,23.24 | 13.21,23.24 v11.81,24.64 13.21,23.24 | v56.26,22.86 v55.24,22.86 55.24,31.11 v55.24,32.38 v53.98,33.66 53.72,33.66 v52.45,33.66 v51.18,32.38
ALARM  (via drill 0.41)
  Top 0.254: v50.59,39.67 U2.53 | RN1.4 76.74,21.84 79.63,21.84 80.14,21.84 J2.1 | D5.C 81.92,27.97 v81.92,29.46
  Bottom 0.254: J2.1 82.17,25.91 | 82.17,25.91 78.11,29.97 70.74,29.97 60.45,29.97 50.8,39.62 v50.59,39.67 | v81.92,29.46 82.17,29.21 82.17,25.91
CMP  (via drill 0.41)
  Top 0.254: C12.2 84.96,43.05 v84.96,42.93 | v80.39,48.26 80.31,48.34 IC7.5 | RN5.3 71.36,56.24 71.37,56.26 70.56,55.57 RN5.5 70.56,52.76 v70.48,52.83
  Bottom 0.254: v84.96,42.93 80.39,47.5 v80.39,48.26 80.39,50.29 77.85,52.83 v70.48,52.83
CTS_B
  Top 0.254: J5.3 51.69,68.07 47.82,64.2 U1.14 45.4,64.2 45.34,64.26
DOG_RESET  (via drill 0.41)
  Top 0.254: U2.52 48.05,40.17 48.39,40.51 48.39,41.27 v47.62,42.04 | v32.64,77.09 32.26,76.71 32.26,73.55 DOGSTAMP.71
  Bottom 0.254: v47.62,42.04 34.8,54.86 34.8,75.82 33.53,77.09 v32.64,77.09
DOG_RX  (via drill 0.41)
  Top 0.254: U2.64 46.11,34.17 43.31,31.37 v43.31,31.11 | v5.71,40.89 3.83,40.89 DOGSTAMP.50
  Bottom 0.254: v43.31,31.11 15.49,31.11 v5.71,40.89
DOG_TX  (via drill 0.41)  (1 unrouted)
  Top 0.254: U2.63 45.85,34.67 43.31,32.13 v42.55,32.13 | v5.71,42.93 3.8,42.93
  Bottom 0.254: v42.55,32.13 16.51,32.13 v5.71,42.93
DTR  (via drill 0.41)
  Top 0.254: U3.13 v73.54,64.52 v73.53,64.52 | v68.96,58.67 68.2,57.91 C7.1 R3.2
  Bottom 0.254: v73.53,64.52 72.77,64.52 72.01,64.52 68.07,60.71 68.07,59.56 v68.96,58.67
GATE_CMD  (via drill 0.41)
  Top 0.254: v77.34,51.56 77.62,51.84 T1.3 | IC7.7 77.02,47.06 v77.34,46.74
  Bottom 0.254: v77.34,46.74 v77.34,51.56
GND  (via drill 0.41)
  Top 0.254: U3.3 78.6,65.52 U3.33 78.61,64.77 v79.12,66.04 | C8.2 84.33,68.58 83.57,69.34 82.93,69.34 v82.42,69.85 | IC1.1 89.51,51.84 89.53,51.82 | v83.95,49.53 PC2.- | IC7.4 79.67,44.12 C2.2 | IC7.4 78.32,41.81 PC1.- | IC7.3 IC7.4 | R3.1 66.29,56.01 67.18,56.9 67.18,58.93 66.29,59.82 C9.2 67.18,61.34 67.18,65.41 v68.58,66.8 68.58,68.71 67.94,69.34 67.94,70.87 C15.2 69.71,71.39 X1.4 71.36,71.39 73.16,69.58 X1.2 | 58.61,61.28 C17.2 | C13.2 46.48,54.86 50.55,54.86 C16.2 51.82,56.01 52.96,54.86 58.8,54.86 | RESET.4 91.21,23.37 90.81,23.37 89.03,25.15 89.03,26.92 89.92,27.81 C11.2 90.04,29.31 RESET.3 89.2,33.78 76.58,33.78 | C3.2 v53.47,24.51 | v53.21,32.38 53.98,32.38 56.39,34.8 60.96,34.8 62.09,33.67 62.88,33.67 65.52,33.67 C5.2 | v53.21,32.38 53.21,34.16 57.99,38.94 U2.32 57.99,43.89 58.29,44.2 58.29,44.45 C6.2 | v53.21,32.38 52.45,32.38 49.66,35.17 U2.62 44.7,35.17 C4.2 | U2.99 60.49,27.65 59.31,28.83 v53.47,28.83 52.45,28.83 51.49,27.87 U2.81 51.49,25.09 C1.2 | R5.2 90.93,55.37 v87.76,55.37 | RN5.4 69.81,56.55 v69.47,56.9 | 73.42,69.6 X1.2 | C14.2 74.79,69.58 X1.2 | C21.2 62.48,49.91 | X3.4 57.8,47.74 X3.2 | C20.2 55.99,49.53 X3.2 | X3.2 56.02,49.54 59.44,52.96
  Top 0.406: U1.4 58.61,61.28 | C17.2 59.82,60.07 59.82,57.15 58.8,56.13 58.8,54.86 58.8,53.59 59.44,52.96 62.48,49.91 63.12,49.28 64.14,49.28 64.9,48.51 64.9,47.24 63.63,45.97 J3.6
  Top 0.813: J4.2 86.87,42.93 C12.1 85.85,45.23 PC2.- | IC1.1 87.02,51.84 85.98,50.8 85.98,49.16 PC2.- | PC2.- 82.68,45.86 82.68,41.91 81.78,41.01 PC1.- 77.97,41.01 77.34,40.39 v76.58,39.62 v76.58,38.61 76.58,33.78 76.58,30.23 72.01,25.65 J1.1 72.01,21.84 71.5,21.34 v53.47,21.34 v52.45,21.34 37.72,21.34 | 2.16,35.01 2.16,39.01 | DOGSTAMP.64 DOGSTAMP.63 DOGSTAMP.62 DOGSTAMP.61 DOGSTAMP.60 DOGSTAMP.59 3.25,59.01 2.16,57.91 2.16,50.04 3.19,49.01 DOGSTAMP.54 DOGSTAMP.53 DOGSTAMP.52 3.67,44.96 3.17,44.96 2.16,43.94 2.16,39.12 2.16,39.01 | DOGSTAMP.49 2.16,39.01 | DOGSTAMP.47 2.16,35.01 | 2.16,35.01 2.16,34.8 2.16,32 3.16,31.01 DOGSTAMP.45 DOGSTAMP.44 DOGSTAMP.43 DOGSTAMP.42 DOGSTAMP.41 | DOGSTAMP.41 | 37.72,21.34 DOGSTAMP.25 37.72,24.89 37.72,25.01 | 37.72,25.01 37.72,31.01 | 37.72,37.01 37.72,31.24 37.72,31.01 | 37.72,47.01 37.72,56.9 37.72,57.01 | 37.72,57.01 37.72,71.01 | 27.72,71.12 22.99,71.12 21.72,72.39 DOGSTAMP.66 DOGSTAMP.65 | DOGSTAMP.69 27.72,71.12 | 27.72,71.12 27.81,71.12 37.72,71.12 37.72,71.01 | DOGSTAMP.1 37.72,71.01 | DOGSTAMP.8 37.72,57.01 | DOGSTAMP.18 37.72,37.01 | 37.72,37.01 37.72,37.08 37.72,46.99 37.72,47.01 | DOGSTAMP.13 37.72,47.01 | DOGSTAMP.24 37.72,25.01 | DOGSTAMP.21 37.72,31.01 | 37.72,21.34 34.67,21.34 33.72,22.29 DOGSTAMP.27 DOGSTAMP.28 DOGSTAMP.29 DOGSTAMP.30 DOGSTAMP.31 DOGSTAMP.32 DOGSTAMP.33 DOGSTAMP.34 DOGSTAMP.35 DOGSTAMP.36 DOGSTAMP.37 13.72,22.48 12.57,21.34 8.51,21.34 7.72,22.13 DOGSTAMP.40 DOGSTAMP.41
  Bottom 0.254: ICSP1.6 76.83,57.4 | 76.83,57.4 76.83,60.45 76.33,60.96 | GROUND.2 v87.76,55.37 87,55.37 83.95,55.37 | 83.95,55.37 81.92,57.4 76.83,57.4 | 83.95,55.37 v83.95,49.53 | v69.47,56.9 69.47,57.66 71.25,59.44 74.3,59.44 75.82,60.96 76.33,60.96 | 76.33,60.96 76.33,61.47 79.12,64.26 v79.12,66.04 79.5,66.04 82.42,68.96 v82.42,69.85 72.9,69.85 69.85,66.8 v68.58,66.8
  Bottom 0.813: v52.45,21.34 v53.47,21.34 v53.47,24.51 53.47,25.02 v53.47,28.83 53.21,29.08 v53.21,32.38 | v76.58,38.61 v76.58,39.62 74.55,41.66 JP1.9 71.63,43.18 65.79,43.18 J3.6
  other vias: 50.29,71.75 52.96,71.75 55.5,73.15 47.88,45.72 59.05,36.2 56.26,39.62 53.72,40.89 50.04,67.82 60.2,58.42 73.66,44.7 62.23,27.3
  pour Bottom (hatched): 0.13,50.16 0.13,20.19 99.95,20.19 99.95,79.88 29.97,79.88 arc-90 0.25,50.16
  pour Top (hatched): 0.13,50.16 0.13,20.19 99.95,20.19 99.95,79.88 29.97,79.88 arc-90 0.25,50.16
ICSP_MISO
  Top 0.254: U2.22 63.94,39.17 64.9,40.13 64.9,45.85 65.66,46.61 67.44,46.61 J3.1
ICSP_MOSI
  Top 0.254: U2.21 64.33,38.67 66.17,40.51 J3.4
ICSP_SCK  (via drill 0.41)
  Top 0.254: U2.20 64.71,38.17 67.44,40.89 v67.44,44.32
  Bottom 0.254: v67.44,44.32 67.44,46.61 J3.3
IDENT  (via drill 0.41)
  Top 0.254: v49.91,38.73 49.48,39.17 U2.54
  Bottom 0.254: J2.2 79.63,27.43 77.6,29.46 70.48,29.46 60.2,29.46 50.93,38.73 v49.91,38.73
LED_USB  (via drill 0.41)
  Top 0.254: D9.C 34.13,77.06 v33.02,75.95 | v5.71,52.96 3.76,52.96 DOGSTAMP.56
  Bottom 0.254: v33.02,75.95 33.02,65.41 20.57,52.96 v5.71,52.96
LED_WIFI  (via drill 0.41)
  Top 0.254: D8.C 41.27,29.5 v41.27,36.07 | v5.84,50.16 5,51.01 DOGSTAMP.55
  Bottom 0.254: v41.27,36.07 14.61,36.07 5.84,44.83 v5.84,50.16
M8RXD  (via drill 0.41)
  Top 0.254: U3.9 75.4,66.58 v74.8,67.18 | v72.77,63.5 72.52,63.25 72.52,61.98 72.16,61.61 RN4.2
  Bottom 0.254: v74.8,67.18 74.8,64.01 74.3,63.5 v72.77,63.5
M8TXD  (via drill 0.41)
  Top 0.254: RN4.1 73.04,61.21 73.04,61.99 v73.53,62.48 | U3.8 76.1,67.85 76.58,68.33 v77.09,68.33
  Bottom 0.254: v77.09,68.33 77.09,64.26 75.31,62.48 v73.53,62.48
MISO2
  Top 0.254: U3.17 76.1,61.69 77.09,60.71 79.63,60.71 80.64,59.69 ICSP1.1
MOSI2
  Top 0.254: U3.16 75.4,61.63 77.09,59.94 78.61,59.94 79.38,59.18 79.38,57.91 78.11,56.64 ICSP1.4
N$1
  Top 0.254: C3.1 58.8,24.51 59.99,25.7 U2.98
N$2
  Top 0.254: IC7.2 IC7.1
N$3
  Top 0.254: U3.1 79.6,69.12 78.87,69.85 78.87,70.23 78.87,70.99 77.85,72.01 R11.1 C14.1 74.81,71.39 X1.3 73.42,71.37
N$4
  Top 0.254: J6.P3 24.64,75.06 24.64,74.8 24.64,74.04 25.27,73.41 25.44,73.41 DOGSTAMP.68
N$5
  Top 0.254: R4.1 79.85,30.64 D5.A
N$6
  Top 0.254: C19.2 56.9,58.36 U1.1
N$7
  Top 0.254: C18.2 50.29,58.04 48.39,59.94 48.03,60.3 U1.18
N$8
  Top 0.254: U1.19 47.74,59.33 48.39,58.67 48.51,58.55 C18.1
N$9
  Top 0.254: C19.1 55.12,57.53 54.74,57.91 54.74,59.69 55.24,60.2 56.29,60.2 U1.3
N$10
  Top 0.254: C13.1 45.97,57.16 U1.20
N$11
  Top 0.254: U1.17 48.45,61.28 C16.1
N$12
  Top 0.254: D7.C 94.45,57.02 R5.1
N$13
  Top 0.254: D8.A 44.23,24.77 R6.1
N$14  (via drill 0.41)
  Top 0.254: D4.C 69.25,27.97 69.25,29.3 v67.82,30.73 | v53.85,44.32 R7.1
  Bottom 0.254: v67.82,30.73 67.82,30.86 66.55,32.13 64.39,32.13 64.01,31.75 60.96,31.75 54.61,38.1 54.61,39.5 54.61,43.56 v53.85,44.32
N$15  (via drill 0.41)
  Top 0.254: v56.39,53.59 52.61,49.82 52.58,49.78 52.58,47.12 52.99,46.7 U2.42 | v61.09,73.91 60.33,74.68 60.33,77.34 D6.C
  Bottom 0.254: v56.39,53.59 59.31,53.59 61.09,55.37 61.09,62.74 v61.09,73.91
N$16
  Top 0.254: D6.A 62.39,77.12 62.36,76.96 R8.2
N$17  (via drill 0.41)
  Top 0.254: J6.P2 25.3,74.45 v25.4,74.42 | DOGSTAMP.67 23.72,74.26 v23.88,74.42
  Bottom 0.254: v25.4,74.42 v23.88,74.42
N$18
  Top 0.254: J6.P1 25.96,75.13 26.42,74.68 30.48,74.68 30.99,75.18 R9.1
N$19
  Top 0.254: J6.P5 23.32,76.66 23.62,76.96 30.61,76.96 R9.2
N$20
  Top 0.254: D9.A R10.1
N$21
  Top 0.254: U2.34 56.99,44.35 R1.1 56,46.09 X3.3 C20.1
N$54
  Top 0.254: RX.A 69.39,61.13 RN4.4
N$55
  Top 0.254: RN4.3 71.36,63.07 TX.A
PWRIN
  Top 0.813: J4.1 87.92,37.85 D1.A
RD+
  Top 0.254: RN2.4 82.86,64.33 82.42,64.77 82.17,65.02 U3.29
RD-
  Top 0.254: RN2.1 82.86,66.73 81.92,65.79 81.65,65.52 U3.30
RESET  (via drill 0.41)
  Top 0.254: RN5.1 72.95,56.97 73.03,58.04 v72.77,58.42 | C7.2 65.41,57.02 65.41,54.61 66.42,53.59 RESET-EN.1 RESET-EN.2 68.33,53.21 68.45,53.34 v69.47,54.36 | C11.1 91.27,26.04 RESET.1 RESET.2 96.22,22.86 v94.11,22.86 | v89.79,22.86 D3.A 87.76,23.54 v87.76,25.65 | U2.30 58.99,41.59 59.31,41.27 61.59,41.27 62.1,41.78 62.1,42.8 | 62.1,42.8 62.1,46.35 J3.5 | v63.25,42.8 62.1,42.8
  Bottom 0.254: v72.77,58.42 72.77,57.66 v69.47,54.36 63.63,48.51 J3.5 | v89.79,22.86 v94.11,22.86 | v87.76,25.65 74.42,38.99 74.42,39.75 73.79,40.39 65.66,40.39 v63.25,42.8
RESET2  (via drill 0.41)
  Top 0.254: U3.24 80.48,62.32 D2.A 82.5,57.4 79.88,57.4 79.38,56.9 79.38,55.37 78.87,54.86 77.34,54.86 76.83,55.37 76.83,57.4 | 76.83,57.4 ICSP1.5 76.83,57.4 | RN5.7 72.26,55.1 v72.26,54.1
  Bottom 0.254: v72.26,54.1 74.3,56.13 74.3,57.4 ICSP1.5
RTS_Y/A
  Top 0.254: U1.6 57.76,63.23 58.04,63.5 58.04,67.56 54.23,71.37 J5.2
RX_A
  Top 0.254: U1.13 47.78,65.17 49.15,66.55 J5.4
RXL
  Top 0.254: U3.10 69.8,66.02 RX.C
S0RX  (via drill 0.41)
  Top 0.254: RN4.7 72.16,59.04 v71.25,58.17 | U2.2 62.19,29.17 61.76,29.17 60.33,30.61 v60.33,33.53
  Bottom 0.254: v71.25,58.17 71.25,57.4 60.33,46.48 v60.33,33.53
S0TX  (via drill 0.41)
  Top 0.254: RN4.8 72.95,59.51 v74.04,58.42 | v61.21,32.64 61.21,30.48 62.02,29.67 U2.3
  Bottom 0.254: v74.04,58.42 73.53,57.91 73.53,57.15 69.98,53.59 69.09,52.7 | 69.09,52.7 68.96,52.58 | v61.21,32.64 61.21,44.83 62.99,46.61 64.14,46.61 64.9,47.37 64.9,48.51 69.09,52.7
SCK2
  Top 0.254: U3.15 74.82,63.52 74.55,63.25 74.55,61.72 77.6,58.67 ICSP1.3
TWI_SCL  (via drill 0.41)
  Top 0.254: v73.79,24.38 74.06,24.66 RN1.2 | v64.39,27.69 64.39,30.73 v64.9,31.24 | v53.72,39.5 52.49,40.73 U2.43 52.49,43.77 52.07,44.2 R7.2
  Bottom 0.254: J1.4 64.39,25.4 64.39,27.43 v64.39,27.69 65.15,28.45 69.98,28.45 73.03,28.45 74.55,26.92 74.55,25.65 74.55,25.15 v73.79,24.38 | v64.9,31.24 60.71,31.24 53.72,38.23 v53.72,39.5
TWI_SDA  (via drill 0.41)
  Top 0.254: RN1.1 73.98,25.46 v73.79,25.65 | v65.66,27.69 65.66,29.97 v66.42,30.73 | v52.45,39.5 51.99,39.96 U2.44
  Bottom 0.254: J1.3 66.93,24.64 65.66,25.91 v65.66,27.69 69.98,27.69 71.75,27.69 v73.79,25.65 | v66.42,30.73 66.17,30.48 60.71,30.48 52.45,38.73 v52.45,39.5
TX_Z/B
  Top 0.254: J5.1 56.77,70.87 58.8,68.83 58.8,62.74 58.29,62.23 56.41,62.23 U1.5
TXL
  Top 0.254: U3.11 71.96,65.52 TX.C
UD+
  Top 0.254: RN2.5 85.66,64.33 86.74,63.25 | 86.74,63.25 87,63.5 87.57,63.5 X2.3 | 86.74,63.25 86.74,59.2 Z2.2
UD-
  Top 0.406: Z1.2 86.76,71.87 87.25,71.37 90.55,68.07 90.55,67.06 89.79,66.29 88.36,66.29 X2.2 85.42,66.73 RN2.8
UGND  (via drill 0.41)
  Top 0.254: U3.28 81.78,64.52 83.44,62.87 C10.2 | v86.74,56.39 86.74,57.66 L1.1
  Top 0.406: C10.2 84.58,62.87 v85.47,61.98 85.47,59.18 85.47,57.91 85.72,57.66 L1.1
  Bottom 0.254: GROUND.1 90.81,56.64 87,56.64 v86.74,56.39
  Bottom 0.406: X2.4 90.55,66.1 90.55,64.26 88.27,61.98 v85.47,61.98
UI_MISO/RXD
  Top 0.254: U2.12 68.19,34.17 69.6,32.77 71.88,32.77 JP1.3
UI_MOSI/TXD
  Top 0.254: U2.13 68.71,34.67 69.34,34.04 JP1.4
UI_SCLK/GPIO3
  Top 0.254: U2.14 65.4,35.17 65.53,35.31 71.88,35.31 JP1.5
UI_SS0/GPIO0
  Top 0.254: U2.15 64.88,35.67 65.79,36.58 69.34,36.58 JP1.6
UI_SS1/GPIO1
  Top 0.254: U2.16 64.49,36.17 66.29,37.97 72.01,37.97 72.39,38.35 JP1.7
UI_SS2/GPIO2
  Top 0.254: U2.17 64.1,36.67 66.55,39.12 69.34,39.12 JP1.8
USBVCC
  Top 0.254: U3.31 80.88,66.02 81.41,66.55 81.41,68.07 81.66,68.33 | F1.1 81.03,70.69 81.03,70.36 81.03,70.31 81.03,68.96 81.66,68.33 | C8.1 81.66,68.33
  Top 0.813: F1.1 78.82,73.28 68.33,73.28 64.39,69.34 64.39,54.61 64.39,52.58 65.43,51.54 75.31,51.54 T1.1
USHIELD
  Top 0.406: Z1.1 90.71,73.41 X2.P$2 X2.P$1 90.71,59.18 Z2.1 88.76,57.88 L1.2
UVCC
  Top 0.813: X2.1 87.11,68.13 84.33,70.87 84.37,71.17 F1.2
VIN  (via drill 0.41)
  Top 0.254: v80.9,42.16 C2.1 81.66,44.32 v81.66,48.77 | PC1.+ 80.9,37.99 v80.9,39.62 | RN5.6 71.25,55.1 71.25,53.59 71.75,53.09 72.77,53.09 73.28,53.59 77.6,53.59 77.6,53.09 77.85,52.83 80.14,52.83 v80.9,52.07
  Top 0.813: PC1.+ 84.76,36.21 D1.C 85.56,35.81 93.6,35.81 93.85,36.07 94.87,37.08 94.87,43.69 91.34,47.22 IC1.3
  Bottom 0.254: v80.9,42.16 v80.9,39.62 | v81.66,48.77 81.66,51.31 v80.9,52.07
VUCAP
  Top 0.254: U3.27 81.27,64.02 C10.1
XT1
  Top 0.254: 58.04,49.8 X3.1 59.31,48.53 | U2.33 57.49,45.63 R1.2 58.17,45.72 59.31,46.86 59.31,48.53 | C21.1 60.31,49.53 59.31,48.53
XT2
  Top 0.254: U3.2 79.1,68.6 78.61,69.09 77.6,70.1 | C15.1 69.73,69.58 X1.1 72.88,67.82 74.17,67.82 75.31,68.96 76.45,68.96 77.6,70.1 | 77.6,70.1 R11.2
Z_CTS  (via drill 0.41)
  Top 0.254: U1.7 51.88,64.2 v51.18,63.5 | v51.18,53.85 51.18,52.58 44.83,46.23 44.83,38.99 45.65,38.17 U2.56
  Bottom 0.254: v51.18,63.5 51.18,61.47 v51.18,53.85
Z_FAST  (via drill 0.41)
  Top 0.254: U1.10 52.01,67.13 v48.39,63.5 | v48.39,53.59 47.37,52.58 43.31,48.51 43.31,38.23 44.86,36.67 U2.59
  Bottom 0.254: v48.39,63.5 48.39,62.48 v48.39,53.59
Z_HDPLX  (via drill 0.41)
  Top 0.254: U1.12 47.23,66.15 v48.13,67.06 | v48.39,52.32 43.81,47.75 43.81,38.48 45.12,37.17 U2.58
  Bottom 0.254: v48.13,67.06 49.4,65.79 49.4,61.21 49.4,53.34 v48.39,52.32
Z_RS485  (via drill 0.41)
  Top 0.254: U1.11 46.68,67.13 v47.62,68.07 | v47.12,53.59 46.61,53.09 42.8,49.28 42.8,37.97 44.6,36.17 U2.60
  Bottom 0.254: v47.62,68.07 47.12,67.56 47.12,62.48 v47.12,53.59
Z_RTS  (via drill 0.41)
  Top 0.254: U1.15 47.14,63.23 47.88,62.48 51.94,62.48 v52.45,62.99 | v52.45,53.59 52.45,52.58 45.34,45.47 45.34,39.24 45.91,38.67 U2.55
  Bottom 0.254: v52.45,62.99 52.45,61.47 v52.45,53.59
Z_RX  (via drill 0.41)
  Top 0.254: U1.8 54.63,65.17 v54.48,65.02 | v54.48,53.34 54.48,52.7 51.49,49.71 51.05,49.28 51.05,44.32 51.49,43.89 U2.45 51.49,37.03 v52.07,36.45 | RN1.3 74.53,23.86 v73.79,23.11
  Bottom 0.254: v54.48,65.02 v54.48,53.34 | v73.79,23.11 75.31,24.64 75.31,27.18 73.53,28.96 70.23,28.96 59.94,28.96 52.45,36.45 v52.07,36.45
Z_TX  (via drill 0.41)
  Top 0.254: U1.16 47.1,62.25 47.37,61.98 v53.47,61.98 | v53.47,52.83 50.99,50.36 50.55,49.91 50.55,44.07 50.99,43.62 U2.46
  Bottom 0.254: v53.47,61.98 v53.47,52.83

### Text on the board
Top: SANDS MOTHERBOARD 001
tSilk: USB | ACT | COMM | ON | POWER | ACT | ALARM | TWI | IDAL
